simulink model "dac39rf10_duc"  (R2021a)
settings: Solver=FixedStepDiscrete  StartTime=0.0  StopTime=4136  RelTol=1e-3
StopFcn:
  | % Get interpolation factor from the L parameter on the DUC subsystem
  | duc = [gcs '/DUC']
  | Lstr = get_param(duc, 'L');
  | L = str2double(erase(Lstr, 'x'));
  | 
  | % Toss out 40*L output samples (40 input sample periods) for startup
  | N_in = size(dac_out,1)/L -40;
  | % Then assume input is bin-centered to the largest power of 2
  | N_in = 2^floor(log2(N_in));
  | % Multiply by L
  | N = N_in*L;
  | 
  | 
  | % Plot 2 channels
  | for ch = 0:1
  | 
  | 
  |     figure(ch+1);
  |     dac = dac_out(:,ch+1);
  |     dac_end = dac(end-N+1:end);
  |     f = [0:N/2];
  | 
  |     dac_fft = fft(dac_end/N*2);
  |     dac_fft = db( dac_fft(1:N/2+1) );
  |     dac_fft = max(dac_fft, -200*ones(N/2+1,1));
  | 
  |     plot(f, dac_fft);
  |     ylim([-150 3]);
  |     yticks([-200:10:0]);
  |     xlim([0 0.5]*N);
  |     xticks([0:0.5/8:0.5]*N);
  |     grid on;
  |     title(['DAC' num2str(ch) ' Output (' num2str(N) ' points)']);
  |     xlabel('Frequency Bin');
  |     ylabel('dBFS');
  | 
  | end
undefined symbols (not defined in the file): j, timearray
libraries: dspmlti4 x64, simulink x5
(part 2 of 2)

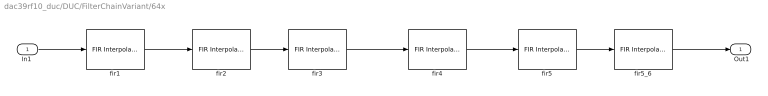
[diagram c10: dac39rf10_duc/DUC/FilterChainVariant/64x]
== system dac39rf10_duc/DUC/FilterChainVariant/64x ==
  "In1 " : Inport
  fir1 : dspmlti4/FIR Interpolation  FilterSource=Dialog parameters  h=[6 0 -19 0 47 0 -100 0 192 0 -342 0 572 0 -914 0 1409 0 -2119 0 3152 0 -4729 0 7420 0 -13334 0 41527 65536 41527 0 -13334 0 7420 0 -4729 0 3152 0 -2119 0 1409 0 -914 0 572 0 -342 0 192 0 -100 0 47 0 -19 0 6 ]*2^-16  L=2  FilterObject=FINTERP  framing=Enforce single-rate processing  outputBufInitCond=0  roundingMode=Round  overflowMode=on  firstCoeffMode=Binary point scaling  firstCoeffWordLength=18  firstCoeffFracLength=16  firstCoeffDataTypeStr=fixdt(1,18,16)  firstCoeffMin=[]  firstCoeffMax=[]  firstCoeffLastDataTypeStr=fixdt(1,18,16)  outputMode=Binary point scaling  outputWordLength=18  outputFracLength=17  outputDataTypeStr=fixdt(1,18,17)  outputMin=[]  outputMax=[]  outputLastDataTypeStr=fixdt(1,18,17)
  fir2 : dspmlti4/FIR Interpolation  FilterSource=Dialog parameters  h=[-12 0 84 0 -336 0 1006 0 -2691 0 10141 16384 10141 0 -2691 0 1006 0 -336 0 84 0 -12 ]*2^-14  L=2  FilterObject=FINTERP  framing=Enforce single-rate processing  outputBufInitCond=0  roundingMode=Round  overflowMode=on  firstCoeffMode=Binary point scaling  firstCoeffWordLength=16  firstCoeffFracLength=14  firstCoeffDataTypeStr=fixdt(1,16,14)  firstCoeffMin=[]  firstCoeffMax=[]  firstCoeffLastDataTypeStr=fixdt(1,16,14)  outputMode=Binary point scaling  outputWordLength=18  outputFracLength=17  outputDataTypeStr=fixdt(1,18,17)  outputMin=[]  outputMax=[]  outputLastDataTypeStr=fixdt(1,18,17)
  fir3 : dspmlti4/FIR Interpolation  FilterSource=Dialog parameters  h=[29 0 -214 0 1209 2048 1209 0 -214 0 29 ]*2^-11  L=2  FilterObject=FINTERP  framing=Enforce single-rate processing  outputBufInitCond=0  roundingMode=Round  overflowMode=on  firstCoeffMode=Binary point scaling  firstCoeffWordLength=13  firstCoeffFracLength=11  firstCoeffDataTypeStr=fixdt(1,13,11)  firstCoeffMin=[]  firstCoeffMax=[]  firstCoeffLastDataTypeStr=fixdt(1,13,11)  outputMode=Binary point scaling  outputWordLength=17  outputFracLength=16  outputDataTypeStr=fixdt(1,17,16)  outputMin=[]  outputMax=[]  outputLastDataTypeStr=fixdt(1,17,16)
  fir4 : dspmlti4/FIR Interpolation  FilterSource=Dialog parameters  h=[3 0 -25 0 150 256 150 0 -25 0 3 ]*2^-8  L=2  FilterObject=FINTERP  framing=Enforce single-rate processing  outputBufInitCond=0  roundingMode=Round  overflowMode=on  firstCoeffMode=Binary point scaling  firstCoeffWordLength=10  firstCoeffFracLength=8  firstCoeffDataTypeStr=fixdt(1,10,8)  firstCoeffMin=[]  firstCoeffMax=[]  firstCoeffLastDataTypeStr=fixdt(1,10,8)  outputMode=Binary point scaling  outputWordLength=17  outputFracLength=16  outputDataTypeStr=fixdt(1,17,16)  outputMin=[]  outputMax=[]  outputLastDataTypeStr=fixdt(1,17,16)
  fir5 : dspmlti4/FIR Interpolation  FilterSource=Dialog parameters  h=[-1 0 9 16 9 0 -1]*2^-4  L=2  FilterObject=FINTERP  framing=Enforce single-rate processing  outputBufInitCond=0  roundingMode=Round  overflowMode=on  firstCoeffMode=Binary point scaling  firstCoeffWordLength=6  firstCoeffFracLength=4  firstCoeffDataTypeStr=fixdt(1,6,4)  firstCoeffMin=[]  firstCoeffMax=[]  firstCoeffLastDataTypeStr=fixdt(1,6,4)  outputMode=Binary point scaling  outputWordLength=16  outputFracLength=15  outputDataTypeStr=fixdt(1,16,15)  outputMin=[]  outputMax=[]  outputLastDataTypeStr=fixdt(1,16,15)
  fir5_6 : dspmlti4/FIR Interpolation  FilterSource=Dialog parameters  h=[-1 0 9 16 9 0 -1]*2^-4  L=2  FilterObject=FINTERP  framing=Enforce single-rate processing  outputBufInitCond=0  roundingMode=Round  overflowMode=on  firstCoeffMode=Binary point scaling  firstCoeffWordLength=6  firstCoeffFracLength=4  firstCoeffDataTypeStr=fixdt(1,6,4)  firstCoeffMin=[]  firstCoeffMax=[]  firstCoeffLastDataTypeStr=fixdt(1,6,4)  outputMode=Binary point scaling  outputWordLength=16  outputFracLength=15  outputDataTypeStr=fixdt(1,16,15)  outputMin=[]  outputMax=[]  outputLastDataTypeStr=fixdt(1,16,15)
  " Out1" : Outport  VectorParamsAs1DForOutWhenUnconnected=off
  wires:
  fir5/1 -> fir5_6/1
  "In1 "/1 -> fir1/1
  fir1/1 -> fir2/1
  fir2/1 -> fir3/1
  fir3/1 -> fir4/1
  fir4/1 -> fir5/1
  fir5_6/1 -> " Out1"/1

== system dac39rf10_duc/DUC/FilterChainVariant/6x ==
  "In1 " : Inport
  fir2 : dspmlti4/FIR Interpolation  FilterSource=Dialog parameters  h=[-12 0 84 0 -336 0 1006 0 -2691 0 10141 16384 10141 0 -2691 0 1006 0 -336 0 84 0 -12 ]*2^-14  L=2  FilterObject=FINTERP  framing=Enforce single-rate processing  outputBufInitCond=0  roundingMode=Round  overflowMode=on  firstCoeffMode=Binary point scaling  firstCoeffWordLength=16  firstCoeffFracLength=14  firstCoeffDataTypeStr=fixdt(1,16,14)  firstCoeffMin=[]  firstCoeffMax=[]  firstCoeffLastDataTypeStr=fixdt(1,16,14)  outputMode=Binary point scaling  outputWordLength=16  outputFracLength=15  outputDataTypeStr=fixdt(1,16,15)  outputMin=[]  outputMax=[]  outputLastDataTypeStr=fixdt(1,16,15)
  fir3x : dspmlti4/FIR Interpolation  FilterSource=Dialog parameters  h=[-38 -38 0 83 117 0 -214 -281 0 464 584 0 -900 -1102 0 1612 1929 0 -2713 -3190 0 4346 5040 0 -6699 -7684 0 10023 11408 0 -14701 -16661 0 21389 24260 0 -31417 -35960 0 48101 56540 0 -82781 -105224 0 215190 432780 524288 432780 215190 0 -105224 -82781 0 56540 48101 0 -35960 -31417 0 24260 21389 0 -16661 -14701 0 11408 10023 0 -7684 -6699 0 5040 4346 0 -3190 -2713 0 1929 1612 0 -1102 -900 0 584 464 0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  L=3  FilterObject=FINTERP  framing=Enforce single-rate processing  outputBufInitCond=0  roundingMode=Round  overflowMode=on  firstCoeffMode=Binary point scaling  firstCoeffWordLength=21  firstCoeffFracLength=19  firstCoeffDataTypeStr=fixdt(1,21,19)  firstCoeffMin=[]  firstCoeffMax=[]  firstCoeffLastDataTypeStr=fixdt(1,21,19)  outputMode=Binary point scaling  outputWordLength=18  outputFracLength=17  outputDataTypeStr=fixdt(1,18,17)  outputMin=[]  outputMax=[]  outputLastDataTypeStr=fixdt(1,18,17)
  " Out1" : Outport  VectorParamsAs1DForOutWhenUnconnected=off
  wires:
  fir2/1 -> " Out1"/1
  fir3x/1 -> fir2/1
  "In1 "/1 -> fir3x/1

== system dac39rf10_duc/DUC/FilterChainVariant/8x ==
  "In1 " : Inport
  fir1 : dspmlti4/FIR Interpolation  FilterSource=Dialog parameters  PrivateCoeffs=0  h=[6 0 -19 0 47 0 -100 0 192 0 -342 0 572 0 -914 0 1409 0 -2119 0 3152 0 -4729 0 7420 0 -13334 0 41527 65536 41527 0 -13334 0 7420 0 -4729 0 3152 0 -2119 0 1409 0 -914 0 572 0 -342 0 192 0 -100 0 47 0 -19 0 6 ]*2^-16  L=2  FilterObject=FINTERP  framing=Enforce single-rate processing  outputBufInitCond=0  roundingMode=Round  overflowMode=on  firstCoeffMode=Binary point scaling  firstCoeffWordLength=18  firstCoeffFracLength=16  firstCoeffDataTypeStr=fixdt(1,18,16)  firstCoeffMin=[]  firstCoeffMax=[]  firstCoeffLastDataTypeStr=fixdt(1,18,16)  outputMode=Binary point scaling  outputWordLength=18  outputFracLength=17  outputDataTypeStr=fixdt(1,18,17)  outputMin=[]  outputMax=[]  outputLastDataTypeStr=fixdt(1,18,17)
  fir2 : dspmlti4/FIR Interpolation  FilterSource=Dialog parameters  PrivateCoeffs=0  h=[-12 0 84 0 -336 0 1006 0 -2691 0 10141 16384 10141 0 -2691 0 1006 0 -336 0 84 0 -12 ]*2^-14  L=2  FilterObject=FINTERP  framing=Enforce single-rate processing  outputBufInitCond=0  roundingMode=Round  overflowMode=on  firstCoeffMode=Binary point scaling  firstCoeffWordLength=16  firstCoeffFracLength=14  firstCoeffDataTypeStr=fixdt(1,16,14)  firstCoeffMin=[]  firstCoeffMax=[]  firstCoeffLastDataTypeStr=fixdt(1,16,14)  outputMode=Binary point scaling  outputWordLength=18  outputFracLength=17  outputDataTypeStr=fixdt(1,18,17)  outputMin=[]  outputMax=[]  outputLastDataTypeStr=fixdt(1,18,17)
  fir3 : dspmlti4/FIR Interpolation  FilterSource=Dialog parameters  PrivateCoeffs=0  h=[29 0 -214 0 1209 2048 1209 0 -214 0 29 ]*2^-11  L=2  FilterObject=FINTERP  framing=Enforce single-rate processing  outputBufInitCond=0  roundingMode=Round  overflowMode=on  firstCoeffMode=Binary point scaling  firstCoeffWordLength=13  firstCoeffFracLength=11  firstCoeffDataTypeStr=fixdt(1,13,11)  firstCoeffMin=[]  firstCoeffMax=[]  firstCoeffLastDataTypeStr=fixdt(1,13,11)  outputMode=Binary point scaling  outputWordLength=16  outputFracLength=15  outputDataTypeStr=fixdt(1,16,15)  outputMin=[]  outputMax=[]  outputLastDataTypeStr=fixdt(1,16,15)
  " Out1" : Outport  VectorParamsAs1DForOutWhenUnconnected=off
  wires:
  fir2/1 -> fir3/1
  fir1/1 -> fir2/1
  "In1 "/1 -> fir1/1
  fir3/1 -> " Out1"/1

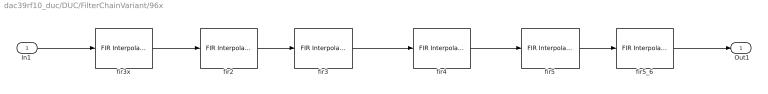
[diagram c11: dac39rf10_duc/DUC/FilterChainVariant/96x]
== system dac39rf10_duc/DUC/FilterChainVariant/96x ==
  "In1 " : Inport
  fir2 : dspmlti4/FIR Interpolation  FilterSource=Dialog parameters  h=[-12 0 84 0 -336 0 1006 0 -2691 0 10141 16384 10141 0 -2691 0 1006 0 -336 0 84 0 -12 ]*2^-14  L=2  FilterObject=FINTERP  framing=Enforce single-rate processing  outputBufInitCond=0  roundingMode=Round  overflowMode=on  firstCoeffMode=Binary point scaling  firstCoeffWordLength=16  firstCoeffFracLength=14  firstCoeffDataTypeStr=fixdt(1,16,14)  firstCoeffMin=[]  firstCoeffMax=[]  firstCoeffLastDataTypeStr=fixdt(1,16,14)  outputMode=Binary point scaling  outputWordLength=18  outputFracLength=17  outputDataTypeStr=fixdt(1,18,17)  outputMin=[]  outputMax=[]  outputLastDataTypeStr=fixdt(1,18,17)
  fir3 : dspmlti4/FIR Interpolation  FilterSource=Dialog parameters  h=[29 0 -214 0 1209 2048 1209 0 -214 0 29 ]*2^-11  L=2  FilterObject=FINTERP  framing=Enforce single-rate processing  outputBufInitCond=0  roundingMode=Round  overflowMode=on  firstCoeffMode=Binary point scaling  firstCoeffWordLength=13  firstCoeffFracLength=11  firstCoeffDataTypeStr=fixdt(1,13,11)  firstCoeffMin=[]  firstCoeffMax=[]  firstCoeffLastDataTypeStr=fixdt(1,13,11)  outputMode=Binary point scaling  outputWordLength=17  outputFracLength=16  outputDataTypeStr=fixdt(1,17,16)  outputMin=[]  outputMax=[]  outputLastDataTypeStr=fixdt(1,17,16)
  fir3x : dspmlti4/FIR Interpolation  FilterSource=Dialog parameters  h=[-38 -38 0 83 117 0 -214 -281 0 464 584 0 -900 -1102 0 1612 1929 0 -2713 -3190 0 4346 5040 0 -6699 -7684 0 10023 11408 0 -14701 -16661 0 21389 24260 0 -31417 -35960 0 48101 56540 0 -82781 -105224 0 215190 432780 524288 432780 215190 0 -105224 -82781 0 56540 48101 0 -35960 -31417 0 24260 21389 0 -16661 -14701 0 11408 10023 0 -7684 -6699 0 5040 4346 0 -3190 -2713 0 1929 1612 0 -1102 -900 0 584 464 0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  L=3  FilterObject=FINTERP  framing=Enforce single-rate processing  outputBufInitCond=0  roundingMode=Round  overflowMode=on  firstCoeffMode=Binary point scaling  firstCoeffWordLength=21  firstCoeffFracLength=19  firstCoeffDataTypeStr=fixdt(1,21,19)  firstCoeffMin=[]  firstCoeffMax=[]  firstCoeffLastDataTypeStr=fixdt(1,21,19)  outputMode=Binary point scaling  outputWordLength=18  outputFracLength=17  outputDataTypeStr=fixdt(1,18,17)  outputMin=[]  outputMax=[]  outputLastDataTypeStr=fixdt(1,18,17)
  fir4 : dspmlti4/FIR Interpolation  FilterSource=Dialog parameters  h=[3 0 -25 0 150 256 150 0 -25 0 3 ]*2^-8  L=2  FilterObject=FINTERP  framing=Enforce single-rate processing  outputBufInitCond=0  roundingMode=Round  overflowMode=on  firstCoeffMode=Binary point scaling  firstCoeffWordLength=10  firstCoeffFracLength=8  firstCoeffDataTypeStr=fixdt(1,10,8)  firstCoeffMin=[]  firstCoeffMax=[]  firstCoeffLastDataTypeStr=fixdt(1,10,8)  outputMode=Binary point scaling  outputWordLength=17  outputFracLength=16  outputDataTypeStr=fixdt(1,17,16)  outputMin=[]  outputMax=[]  outputLastDataTypeStr=fixdt(1,17,16)
  fir5 : dspmlti4/FIR Interpolation  FilterSource=Dialog parameters  h=[-1 0 9 16 9 0 -1]*2^-4  L=2  FilterObject=FINTERP  framing=Enforce single-rate processing  outputBufInitCond=0  roundingMode=Round  overflowMode=on  firstCoeffMode=Binary point scaling  firstCoeffWordLength=6  firstCoeffFracLength=4  firstCoeffDataTypeStr=fixdt(1,6,4)  firstCoeffMin=[]  firstCoeffMax=[]  firstCoeffLastDataTypeStr=fixdt(1,6,4)  outputMode=Binary point scaling  outputWordLength=16  outputFracLength=15  outputDataTypeStr=fixdt(1,16,15)  outputMin=[]  outputMax=[]  outputLastDataTypeStr=fixdt(1,16,15)
  fir5_6 : dspmlti4/FIR Interpolation  FilterSource=Dialog parameters  h=[-1 0 9 16 9 0 -1]*2^-4  L=2  FilterObject=FINTERP  framing=Enforce single-rate processing  outputBufInitCond=0  roundingMode=Round  overflowMode=on  firstCoeffMode=Binary point scaling  firstCoeffWordLength=6  firstCoeffFracLength=4  firstCoeffDataTypeStr=fixdt(1,6,4)  firstCoeffMin=[]  firstCoeffMax=[]  firstCoeffLastDataTypeStr=fixdt(1,6,4)  outputMode=Binary point scaling  outputWordLength=16  outputFracLength=15  outputDataTypeStr=fixdt(1,16,15)  outputMin=[]  outputMax=[]  outputLastDataTypeStr=fixdt(1,16,15)
  " Out1" : Outport  VectorParamsAs1DForOutWhenUnconnected=off
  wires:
  fir5_6/1 -> " Out1"/1
  fir4/1 -> fir5/1
  fir3/1 -> fir4/1
  fir2/1 -> fir3/1
  fir3x/1 -> fir2/1
  "In1 "/1 -> fir3x/1
  fir5/1 -> fir5_6/1
